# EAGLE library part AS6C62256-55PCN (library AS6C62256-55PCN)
Alliance Memory AS6C62256-55PCN SRAM Memory, 256kbit, 2.7 5.5 V, 55ns 28-Pin PDIP Source: Datasheet
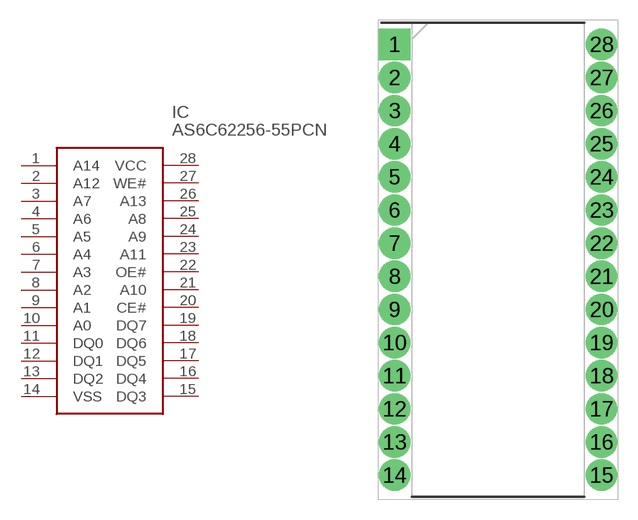
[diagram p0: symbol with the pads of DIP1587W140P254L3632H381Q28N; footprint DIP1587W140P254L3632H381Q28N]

Designator prefix IC

## AS6C62256-55PCN (Description: Alliance Memory AS6C62256-55PCN SRAM Memory, 256kbit, 2.7 5.5 V, 55ns 28-Pin PDIP; Height: 3.81mm; Manufacturer_Name: Alliance Memory; Manufacturer_Part_Number: AS6C62256-55PCN; Mouser_Part_Number: 913-AS6C62256-55PCN; Mouser_Price-Stock: https://www.mouser.co.uk/ProductDetail/Alliance-Memory/AS6C62256-55PCN?qs=LD2UibpCYJqgbIupMJnGTQ%3D%3D)  [DIP1587W140P254L3632H381Q28N]
1  A14  in
2  A12  in
3  A7  in
4  A6  in
5  A5  in
6  A4  in
7  A3  in
8  A2  in
9  A1  in
10  A0  in
11  DQ0
12  DQ1
13  DQ2
14  VSS  pwr
15  DQ3
16  DQ4
17  DQ5
18  DQ6
19  DQ7
20  CE#  in
21  A10  in
22  OE#  in
23  A11  in
24  A9  in
25  A8  in
26  A13  in
27  WE#  in
28  VCC  pwr

## Footprint DIP1587W140P254L3632H381Q28N (pad centres in mm)
AS6C62256
drill 1.597 pad 1.997 square: 1 -7.935,16.51
drill 1.597 pad 1.997: 2 -7.935,13.97; 3 -7.935,11.43; 4 -7.935,8.89; 5 -7.935,6.35; 6 -7.935,3.81; 7 -7.935,1.27; 8 -7.935,-1.27; 9 -7.935,-3.81; 10 -7.935,-6.35; 11 -7.935,-8.89; 12 -7.935,-11.43; 13 -7.935,-13.97; 14 -7.935,-16.51; 15 7.935,-16.51; 16 7.935,-13.97; 17 7.935,-11.43; 18 7.935,-8.89; 19 7.935,-6.35; 20 7.935,-3.81; 21 7.935,-1.27; 22 7.935,1.27; 23 7.935,3.81; 24 7.935,6.35; 25 7.935,8.89; 26 7.935,11.43; 27 7.935,13.97; 28 7.935,16.51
